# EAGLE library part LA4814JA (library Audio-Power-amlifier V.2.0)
The LA4814JA buili-in the power amplifier circuit capable of low-voltage (2.7V and up) operation and has additionally a standby function to reduce the current drain. It is a power amplifier IC optimal for speaker drive used in battery-driven portable equipment and other such products.
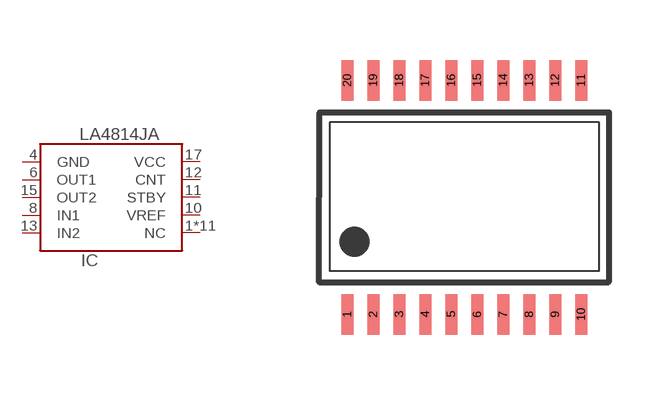
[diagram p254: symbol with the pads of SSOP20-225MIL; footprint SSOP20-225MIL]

Designator prefix IC

## LA4814JA  [SSOP20-225MIL]
1  NC  nc
2  NC  nc
3  NC  nc
4  GND  pwr
5  NC  nc
6  OUT1  out
7  NC  nc
8  IN1  in
9  NC  nc
10  VREF
11  STBY  in
12  CNT
13  IN2  in
14  NC  nc
15  OUT2  out
16  NC  nc
17  VCC  pwr
18  NC  nc
19  NC  nc
20  NC  nc

## Footprint SSOP20-225MIL (pad centres in mm)
Small Shrink Outline Package 225mil SANYO Semiconduktor
smd 0.3 x 1.016: 1 -2.925,-2.925; 2 -2.275,-2.925; 3 -1.625,-2.925; 4 -0.975,-2.925; 5 -0.325,-2.925; 6 0.325,-2.925; 7 0.975,-2.925; 8 1.625,-2.925; 9 2.275,-2.925; 10 2.925,-2.925; 11 2.925,2.925; 12 2.275,2.925; 13 1.625,2.925; 14 0.975,2.925; 15 0.325,2.925; 16 -0.325,2.925; 17 -0.975,2.925; 18 -1.625,2.925; 19 -2.275,2.925; 20 -2.925,2.925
